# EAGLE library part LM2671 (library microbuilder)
LM2671 High Efficiency 500mA Switching Step-Down Voltage Regulator. 6.5-40V Input. 3.3V SOIC-8: Digikey LM2671M-3.3-ND
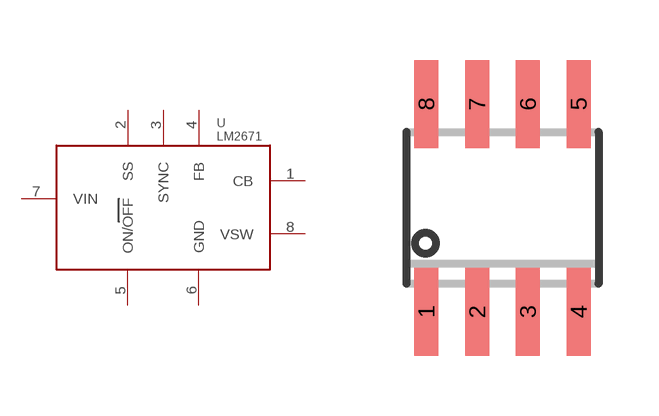
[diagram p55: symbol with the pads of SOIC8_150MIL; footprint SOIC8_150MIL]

Designator prefix U

## LM2671  [SOIC8_150MIL]
1  CB
2  SS
3  SYNC
4  FB
5  ON/OFF
6  GND
7  VIN
8  VSW

## Footprint SOIC8_150MIL (pad centres in mm)
Small Outline IC - 150mil Wide
smd 0.6 x 2.2: 1 -1.905,-2.6; 2 -0.635,-2.6; 3 0.635,-2.6; 4 1.905,-2.6; 5 1.905,2.6; 6 0.635,2.6; 7 -0.635,2.6; 8 -1.905,2.6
